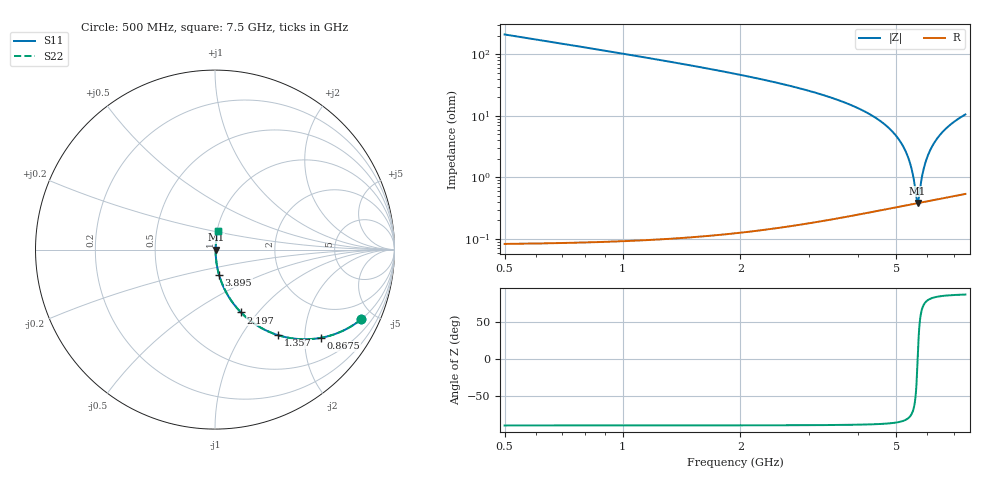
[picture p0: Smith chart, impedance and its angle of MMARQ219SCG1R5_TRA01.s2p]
! MMARQ219SCG1R5_TRA01  S-PARAMETER MODEL  ( General Type )
! Model Generated by TAIYO YUDEN Corporation (http://www.ty-top.com)
! Version 1.0
! TAIYO YUDEN Control No. 180601
! Copyright(c) 2018 TAIYO YUDEN CO.,LTD. All Rights Reserved.
! Product Description (link to TY-COMPAS)
! https://ds.yuden.co.jp/TYCOMPAS/or/detail?pn=MMARQ219SCG1R5BTRA01&u=M
! Products Name : Multilayer Ceramic Capacitors
! Characteristics :
!  Capacitance : 1.5 pF , Rated Voltage : 250V , TCC : CG / C0G
!  Case Size : 2.0 x 1.25 / 0.079 x 0.049 [mm/inch] , Thickness : 0.85 / 0.033 [mm/inch]
!  (Conditions: Temperature = 25 degC , DC Bias Current/Voltage = 0A / 0V)
! External Node Assignments :
!  1  o---| |---o  2
! GND o---------o GND
! Frequency Range : 500MHz  -  7500MHz  [ 401 STEP ]
# MHz S RI R 50
! Freq[MHz].  S11 Real  S11 Imag  S21 Real  S21 Imag  S12 Real  S12 Imag  S22 Real  S22 Imag
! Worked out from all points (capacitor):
!   401 points, 500 MHz to 7.5 GHz, reference 50 ohm
!   read as one part in series: C = 1.5 pF near 535 MHz
!   lowest |Z| = 383 mohm at 5.662 GHz (marker M1)
!   series resonance near 5.665 GHz, so ESL is about 530 pH
!   S11 on the Smith chart (normalised r, x): 500 MHz: 1.00, -4.21; 867.5 MHz: 1.00, -2.39; 1.357 GHz: 1.00, -1.47; 2.197 GHz: 1.00, -0.82; 3.895 GHz: 1.00, -0.29; 7.5 GHz: 1.01, +0.21
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500  0.8159 -0.3873  0.1841 0.3873  0.1841 0.3873  0.8159 -0.3873
867.5  0.5879 -0.4918  0.4121 0.4918  0.4121 0.4918  0.5879 -0.4918
1357.5  0.3519 -0.4769  0.6481 0.4769  0.6481 0.4769  0.3519 -0.4769
1672.5  0.2514 -0.4329  0.7486 0.4329  0.7486 0.4329  0.2514 -0.4329
2197.5  0.1446 -0.3501  0.8554 0.3501  0.8554 0.3501  0.1446 -0.3501
2845  0.0733 -0.2576  0.9267 0.2576  0.9267 0.2576  0.0733 -0.2576
3895  0.0224 -0.1397  0.9776 0.1397  0.9776 0.1397  0.0224 -0.1397
4000  0.0196 -0.1297  0.9804 0.1297  0.9804 0.1297  0.0196 -0.1297
4700  0.00786 -0.0693  0.9921 0.0693  0.9921 0.0693  0.00786 -0.0693
5172.5  0.00454 -0.0337  0.9955 0.0337  0.9955 0.0337  0.00454 -0.0337
5312.5  0.00409 -0.0238  0.9959 0.0238  0.9959 0.0238  0.00409 -0.0238
5435  0.00386 -0.0153  0.9961 0.0153  0.9961 0.0153  0.00386 -0.0153
5522.5  0.00378 -0.00943  0.9962 0.00943  0.9962 0.00943  0.00378 -0.00943
5627.5  0.00379 -0.00247  0.9962 0.00247  0.9962 0.00247  0.00379 -0.00247
5662.5  0.00381 -0.000181  0.9962 0.000181  0.9962 0.000181  0.00381 -0.000181
5697.5  0.00385 0.00209  0.9962 -0.00209  0.9962 -0.00209  0.00385 0.00209
5837.5  0.00408 0.0111  0.9959 -0.0111  0.9959 -0.0111  0.00408 0.0111
5942.5  0.00436 0.0176  0.9956 -0.0176  0.9956 -0.0176  0.00436 0.0176
6117.5  0.005 0.0283  0.995 -0.0283  0.995 -0.0283  0.005 0.0283
6345  0.00614 0.0418  0.9939 -0.0418  0.9939 -0.0418  0.00614 0.0418
6835  0.00963 0.0691  0.9904 -0.0691  0.9904 -0.0691  0.00963 0.0691
7500  0.0162 0.1032  0.9838 -0.1032  0.9838 -0.1032  0.0162 0.1032
